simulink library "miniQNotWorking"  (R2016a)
settings: Solver=VariableStepAuto  StartTime=0.0  StopTime=10.0  RelTol=1e-3
undefined symbols (not defined in the file or in its folder): bin2dec, debug_dd, DiscIntNeverNeededParam, flipLeft, flipRight, maxRawSensors, minRawSensors, sampleTime_dd
libraries: simulink x4, arduinolib x4

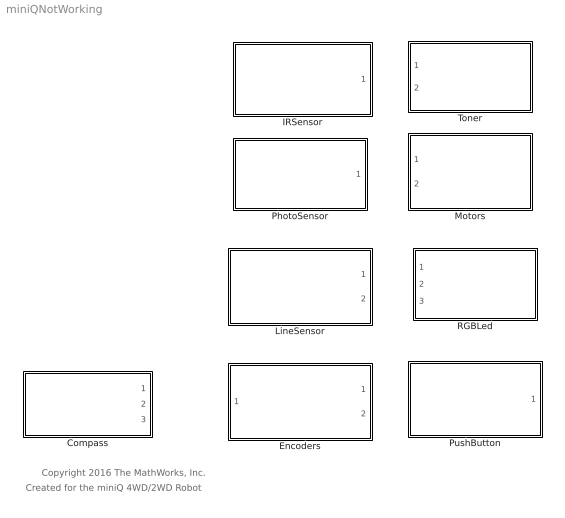
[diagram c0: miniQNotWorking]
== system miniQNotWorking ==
  note: Copyright 2016 The MathWorks, Inc.
  note: Created for the miniQ 4WD/2WD Robot
  Compass : Subsystem  TreatAsAtomicUnit=on
  Encoders : Subsystem
  IRSensor : Subsystem
  LineSensor : Subsystem
  Motors : Subsystem
  PhotoSensor : Subsystem
  PushButton : Subsystem
  RGBLed : Subsystem
  Toner : Subsystem

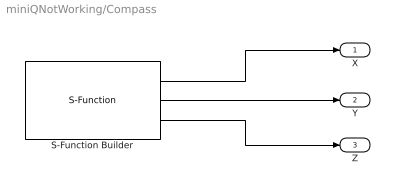
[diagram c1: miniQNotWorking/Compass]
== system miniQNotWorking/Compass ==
  S-Function Builder : S-Function  InitFcn=try, set_param(gcb,'FunctionName','HMC5883L'), end  FunctionName=HMC5883L  Parameters=sampleTime_dd  SFunctionModules=HMC5883L_wrapper  SFunctionDeploymentMode=off  EnableBusSupport=off
  X : Outport
  Y : Outport  Port=2
  Z : Outport  Port=3
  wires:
  S-Function Builder/1 -> X/1
  S-Function Builder/2 -> Y/1
  S-Function Builder/3 -> Z/1

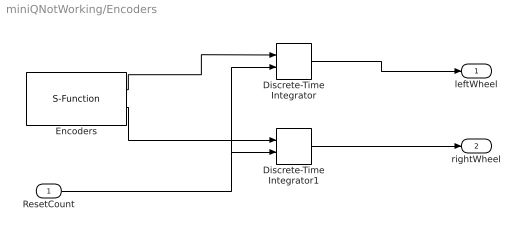
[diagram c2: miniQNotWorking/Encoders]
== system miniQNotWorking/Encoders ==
  ResetCount : Inport
  Discrete-Time Integrator : DiscreteIntegrator  IntegratorMethod=Accumulation: Forward Euler  gainval=1  ExternalReset=rising  InitialConditionSetting=State (most efficient)  SampleTime=-1  ICPrevOutput=DiscIntNeverNeededParam  ICPrevScaledInput=DiscIntNeverNeededParam
  Discrete-Time Integrator1 : DiscreteIntegrator  IntegratorMethod=Accumulation: Forward Euler  gainval=1  ExternalReset=rising  InitialConditionSetting=State (most efficient)  SampleTime=-1  ICPrevOutput=DiscIntNeverNeededParam  ICPrevScaledInput=DiscIntNeverNeededParam
  Encoders : S-Function  InitFcn=try, set_param(gcb,'FunctionName','Encoders'), end  FunctionName=Encoders  Parameters=sampleTime_dd,boolean(debug_dd)  SFunctionModules=Encoders_wrapper  SFunctionDeploymentMode=off  EnableBusSupport=off
  leftWheel : Outport
  rightWheel : Outport  Port=2
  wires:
  Encoders/1 -> Discrete-Time Integrator/1
  Encoders/2 -> Discrete-Time Integrator1/1
  Discrete-Time Integrator/1 -> leftWheel/1
  Discrete-Time Integrator1/1 -> rightWheel/1
  ResetCount/1 -> Discrete-Time Integrator1/2, Discrete-Time Integrator/2

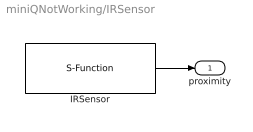
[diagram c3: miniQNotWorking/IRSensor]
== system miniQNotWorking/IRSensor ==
  IRSensor : S-Function  InitFcn=try, set_param(gcb,'FunctionName','IRSensor'), end  FunctionName=IRSensor  Parameters=sampleTime_dd,boolean(debug_dd)  SFunctionModules=IRSensor_wrapper  SFunctionDeploymentMode=off  EnableBusSupport=off
  proximity : Outport
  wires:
  IRSensor/1 -> proximity/1

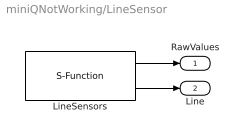
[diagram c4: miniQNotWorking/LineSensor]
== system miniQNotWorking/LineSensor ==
  LineSensors : S-Function  InitFcn=try, set_param(gcb,'FunctionName','LineSensor'), end  FunctionName=LineSensor  Parameters=sampleTime_dd,boolean(debug_dd),uint16(maxRawSensors),uint16(minRawSensors)  SFunctionModules=LineSensor_wrapper  SFunctionDeploymentMode=off  EnableBusSupport=off
  RawValues : Outport
  Line : Outport  Port=2
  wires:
  LineSensors/1 -> RawValues/1
  LineSensors/2 -> Line/1

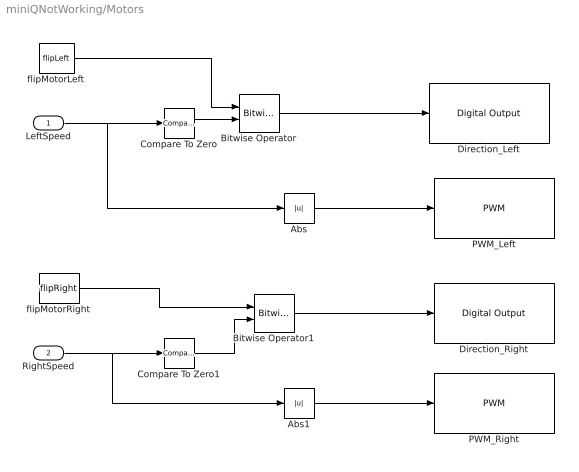
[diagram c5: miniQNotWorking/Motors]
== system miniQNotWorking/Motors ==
  LeftSpeed : Inport
  RightSpeed : Inport  Port=2
  Abs : Abs  OutDataTypeStr=uint8
  Abs1 : Abs  OutDataTypeStr=uint8
  Bitwise Operator : simulink/Logic and Bit Operations/Bitwise Operator  logicop=OR  UseBitMask=off  NumInputPorts=2  BitMask=bin2dec('11011001')  BitMaskRealWorld=Stored Integer
  Bitwise Operator1 : simulink/Logic and Bit Operations/Bitwise Operator  logicop=OR  UseBitMask=off  NumInputPorts=2  BitMask=bin2dec('11011001')  BitMaskRealWorld=Stored Integer
  Compare To Zero : simulink/Logic and Bit Operations/Compare To Zero  relop=<  OutDataTypeStr=boolean
  Compare To Zero1 : simulink/Logic and Bit Operations/Compare To Zero  relop=<  OutDataTypeStr=boolean
  Direction_Left : arduinolib/Digital Output  pinNumber=12  blockPlatform=arduino
  Direction_Right : arduinolib/Digital Output  pinNumber=7  blockPlatform=arduino
  PWM_Left : arduinolib/PWM  pinNumber=5  blockPlatform=arduino
  PWM_Right : arduinolib/PWM  pinNumber=6  blockPlatform=arduino
  flipMotorLeft : Constant  Value=flipLeft  OutDataTypeStr=boolean
  flipMotorRight : Constant  Value=flipRight  OutDataTypeStr=boolean
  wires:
  Compare To Zero/1 -> Bitwise Operator/2
  Abs/1 -> PWM_Left/1
  Abs1/1 -> PWM_Right/1
  flipMotorLeft/1 -> Bitwise Operator/1
  LeftSpeed/1 -> Abs/1, Compare To Zero/1
  flipMotorRight/1 -> Bitwise Operator1/1
  Compare To Zero1/1 -> Bitwise Operator1/2
  Bitwise Operator1/1 -> Direction_Right/1
  RightSpeed/1 -> Abs1/1, Compare To Zero1/1
  Bitwise Operator/1 -> Direction_Left/1

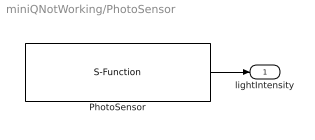
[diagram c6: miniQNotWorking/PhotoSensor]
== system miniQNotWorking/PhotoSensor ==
  PhotoSensor : S-Function  InitFcn=try, set_param(gcb,'FunctionName','PhotoSensor'), end  FunctionName=PhotoSensor  Parameters=sampleTime_dd,boolean(debug_dd)  SFunctionModules=PhotoSensor_wrapper  SFunctionDeploymentMode=off  EnableBusSupport=off
  lightIntensity : Outport
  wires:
  PhotoSensor/1 -> lightIntensity/1

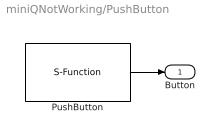
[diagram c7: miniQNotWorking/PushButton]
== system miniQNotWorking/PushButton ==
  PushButton : S-Function  InitFcn=try, set_param(gcb,'FunctionName','PushButton'), end  FunctionName=PushButton  Parameters=sampleTime_dd,boolean(debug_dd)  SFunctionModules=PushButton_wrapper  SFunctionDeploymentMode=off  EnableBusSupport=off
  Button : Outport
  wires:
  PushButton/1 -> Button/1

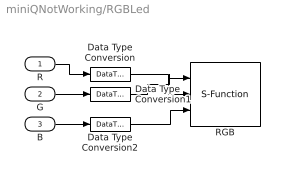
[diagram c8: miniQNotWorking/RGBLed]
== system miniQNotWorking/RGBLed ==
  R : Inport
  G : Inport  Port=2
  B : Inport  Port=3
  Data Type Conversion : DataTypeConversion  OutDataTypeStr=uint8
  Data Type Conversion1 : DataTypeConversion  OutDataTypeStr=uint8
  Data Type Conversion2 : DataTypeConversion  OutDataTypeStr=uint8
  RGB : S-Function  InitFcn=try, set_param(gcb,'FunctionName','RGB'), end  FunctionName=RGB  SFunctionModules=RGB_wrapper  SFunctionDeploymentMode=off  EnableBusSupport=off
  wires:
  B/1 -> Data Type Conversion2/1
  G/1 -> Data Type Conversion1/1
  R/1 -> Data Type Conversion/1
  Data Type Conversion/1 -> RGB/2
  Data Type Conversion1/1 -> RGB/1
  Data Type Conversion2/1 -> RGB/3

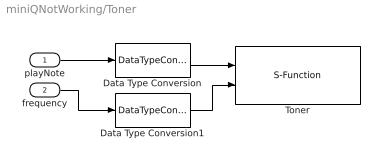
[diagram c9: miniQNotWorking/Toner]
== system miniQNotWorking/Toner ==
  playNote : Inport
  frequency : Inport  Port=2
  Data Type Conversion : DataTypeConversion  OutDataTypeStr=boolean
  Data Type Conversion1 : DataTypeConversion  OutDataTypeStr=uint16
  Toner : S-Function  InitFcn=try, set_param(gcb,'FunctionName','Toner'), end  FunctionName=Toner  SFunctionModules=Toner_wrapper  SFunctionDeploymentMode=off  EnableBusSupport=off
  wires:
  playNote/1 -> Data Type Conversion/1
  Data Type Conversion/1 -> Toner/1
  Data Type Conversion1/1 -> Toner/2
  frequency/1 -> Data Type Conversion1/1
